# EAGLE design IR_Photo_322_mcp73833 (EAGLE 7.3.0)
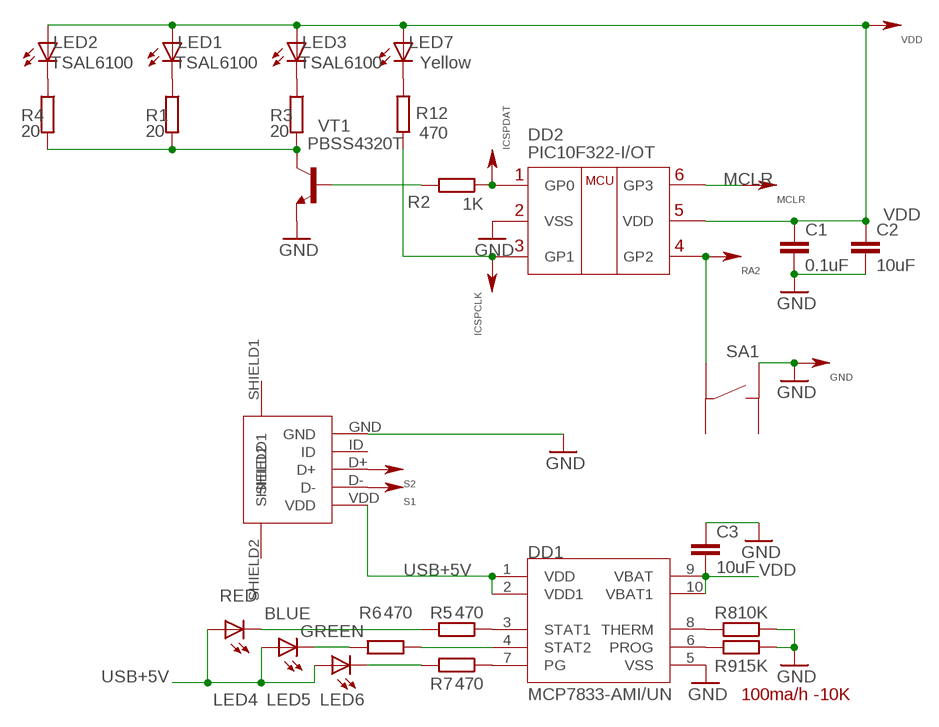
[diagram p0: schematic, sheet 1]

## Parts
C1  0.1uF  C-EUC0805  [C0805]
C2  10uF  C-EUC0805  [C0805]
C3  10uF  C-EUC0805  [C0805]
DD1  MCP7833-AMI/UN  MCP73833  [MSOP10]
DD2  PIC10F322-I/OT  PIC10F20XSOT23-6  [SOT23-6]
GND  1-PINSMD  [1-PINSMD]
ICSPCLK  1-PINSMD  [1-PINSMD]
ICSPDAT  1-PINSMD  [1-PINSMD]
LED1  TSAL6100  LEDNO_HOLE_MIR  [LED_NO_HOLE_MIR]
LED2  TSAL6100  LEDNO_HOLE_MIR  [LED_NO_HOLE_MIR]
LED3  TSAL6100  LEDNO_HOLE_MIR  [LED_NO_HOLE_MIR]
LED4  RED  LEDCHIPLED_1206  [CHIPLED_1206]
LED5  BLUE  LEDCHIPLED_1206  [CHIPLED_1206]
LED6  GREEN  LEDCHIPLED_1206  [CHIPLED_1206]
LED7  Yellow  LEDCHIPLED_1206  [CHIPLED_1206]
MCLR  1-PINSMD  [1-PINSMD]
R1  20  R-EU_R0805  [R0805]
R2  1K  R-EU_R0603  [R0603]
R3  20  R-EU_R0805  [R0805]
R4  20  R-EU_R0805  [R0805]
R5  470  R-EU_R0603  [R0603]
R6  470  R-EU_R0603  [R0603]
R7  470  R-EU_R0603  [R0603]
R8  10K  R-EU_R0603  [R0603]
R9  15K  R-EU_R0603  [R0603]
R12  470  R-EU_R0603  [R0603]
RA2  1-PINSMD  [1-PINSMD]
S1  1-PINSMD  [1-PINSMD]
S2  1-PINSMD  [1-PINSMD]
SA1  TACKT_BUTTONIIT-1102S  [IIT-1102S]
U$8  USB-MICRO  [USB-MICRO-SMD]
VDD  1-PINSMD  [1-PINSMD]
VT1  PBSS4320T  PBSS4320T-NPN-SOT23-BEC  [SOT23-BEC]

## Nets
GND: C1.2 C2.2 C3.1 DD1.5(VSS) DD2.2(VSS) GND.1(S) R8.1 R9.1 SA1.SR U$8.GND VT1.E
ICSPDAT: DD2.1(GP0) ICSPDAT.1(S) R2.1
MCLR: DD2.6(GP3) MCLR.1(S)
N$1: LED1.CATOD(C) R1.1
N$2: LED7.C R12.2
N$4: LED2.CATOD(C) R4.1
N$5: R2.2 VT1.B
N$6: R1.2 R3.2 R4.2 VT1.C
N$8: DD2.4(GP2) RA2.1(S) SA1.SSR
N$9: LED3.CATOD(C) R3.1
N$10: DD1.3(STAT1) R5.1
N$11: DD1.7(PG) R7.1
N$12: S1.1(S) U$8.D-
N$13: DD1.6(PROG) R9.2
N$14: LED4.C R5.2
N$15: LED5.C R6.2
N$16: DD1.4(STAT2) R6.1
N$17: LED6.C R7.2
N$18: DD1.8(THERM) R8.2
N$19: S2.1(S) U$8.D+
N$24: DD2.3(GP1) ICSPCLK.1(S) R12.1
USB+5V: DD1.1(VDD) DD1.2(VDD1) LED4.A LED5.A LED6.A U$8.VDD
VDD: C1.1 C2.1 C3.2 DD1.9(VBAT) DD1.10(VBAT1) DD2.5(VDD) LED1.ANOD(A) LED2.ANOD(A) LED3.ANOD(A) LED7.A VDD.1(S)
Unconnected: SA1.SL SA1.SSL U$8.ID U$8.SHIELD1 U$8.SHIELD2

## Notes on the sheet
- 100ma/h -10K

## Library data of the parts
C1-C3 = resistors:C-EU: CAPACITOR, European symbol
DD1 = power:MCP73833
DD2 = Microchip:PIC10F20X
GND ICSPCLK ICSPDAT MCLR RA2 S1 S2 VDD = connectors:1-PIN
LED1-LED7 = led:LED: LED
R1-R9 R12 = resistors:R-EU_: RESISTOR, European symbol
SA1 = button:TACKT_BUTTON
U$8 = connectors:USB-MICRO
VT1 = Tranzistors:*-NPN-: NPN Transistror BF959 corrected 2008.03.06

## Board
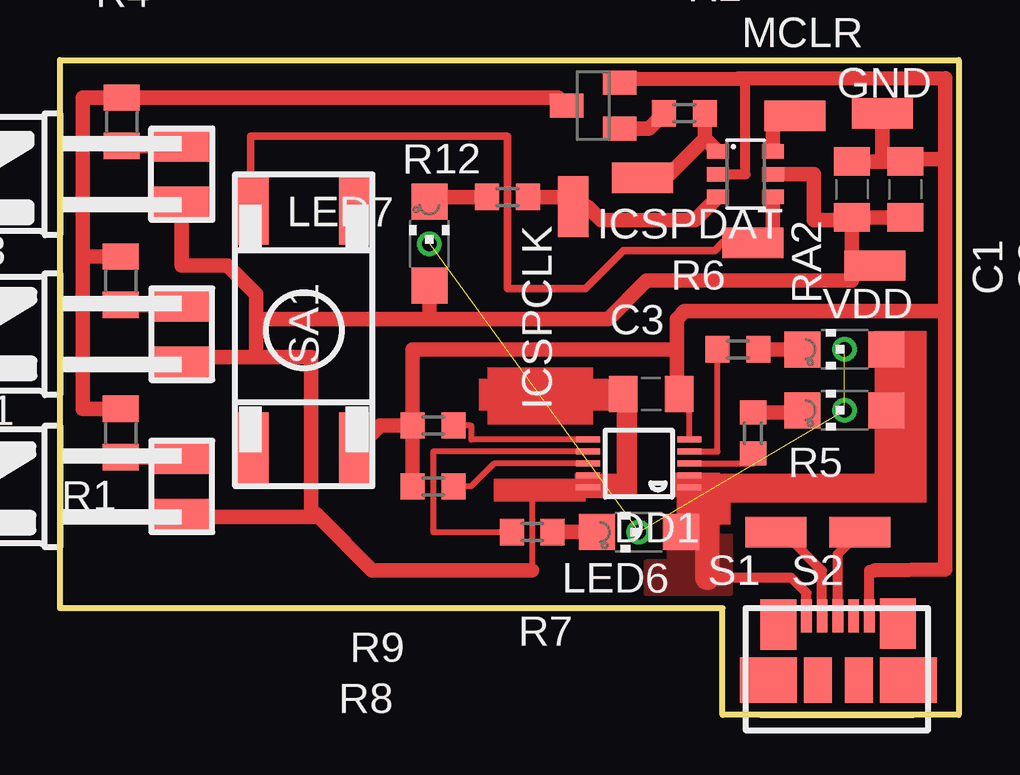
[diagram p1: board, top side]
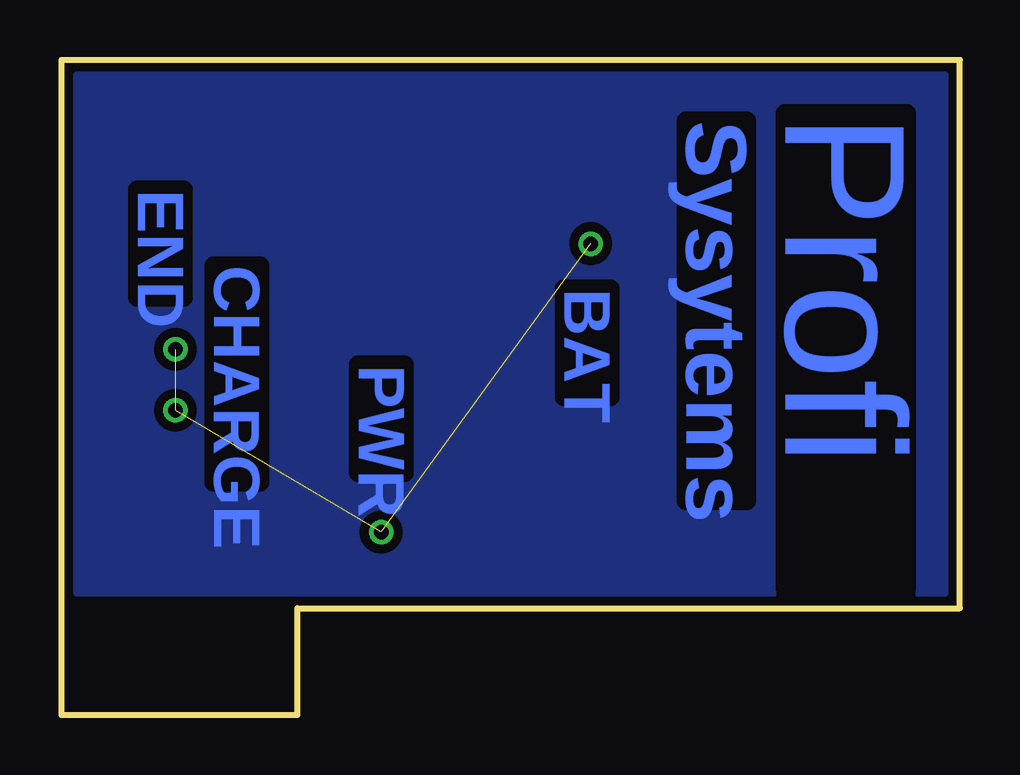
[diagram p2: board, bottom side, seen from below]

Size 37.47 x 27.3 mm. Coordinates in mm from the lower left corner, seen from the top.
Outline: 37.45,4.45 37.45,27.29 0,27.29 0,4.45
Outline: 0,4.45 27.62,4.45 27.62,0 37.47,0 37.47,27.3 0,27.3 0,4.45
Copper layers (1*16): Top 0.035mm / dielectric 1.5mm / Bottom 0.035mm
Design rules "default *": minimum track width 4mil, minimum drill 2mil, track to track 15mil, track to pad 8mil, pad to pad 8mil, via to via 8mil, smd to smd 8mil, copper to edge 10mil, drill to drill 20mil, minimum pad ring 4mil, minimum via ring 4mil, stop-mask expansion 4mil, vias tented up to drill 0mil, thermal gap 10mil

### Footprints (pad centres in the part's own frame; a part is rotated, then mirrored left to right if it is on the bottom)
C0805 = smd 1.2 x 1.5: 1 -1.167,0; 2 1.167,0
MSOP10 = smd 0.25 x 1: 1 -1,-2.113; 2 -0.5,-2.113; 3 0,-2.113; 4 0.5,-2.113; 5 1,-2.113; 6 1,2.113; 7 0.5,2.113; 8 0,2.113; 9 -0.5,2.113; 10 -1,2.113
SOT23-6 = smd 0.6 x 0.9: 1 -0.95,-1.15; 2 0,-1.15; 3 0.95,-1.15; 4 0.95,1.15; 5 0,1.15; 6 -0.95,1.15
1-PINSMD = smd 2.54 x 1.27: 1 0,0
LED_NO_HOLE_MIR = smd 2.5 x 1.5: ANOD 0,2.54; CATOD 0,0
CHIPLED_1206 = smd 1.5 x 1.5: A 0,-1.75; C 0,1.75
R0805 = smd 1.1 x 1.5: 1 -1.009,0; 2 1.009,0
R0603 = smd 1 x 1.1: 1 -0.85,0; 2 0.85,0
IIT-1102S = smd 3 x 1.5: SL 10.001,0; SR 0,0; SSL 0,4.445; SSR 10.001,4.445
USB-MICRO-SMD = smd 1.38 x 0.45: D+ 0,-1.627; D- 0,-0.972; GND 0,-2.937; ID 0,-2.282; VDD 0,-0.318 | smd 2.1 x 1.5: P$1 -0.318,-4.128; P$2 -0.357,0.853 | smd 1.9 x 1.175: P$5 -2.679,-2.5; P$6 -2.679,-0.794 | smd 1.9 x 2.375: SHIELD1 -2.679,1.27; SHIELD2 -2.679,-4.564
SOT23-BEC = smd 1 x 1.4: B -0.95,-1.1; C 0,1.1; E 0.95,-1.1

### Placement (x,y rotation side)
C1  33.02,21.91 90 top
C2  35.24,21.91 90 top
C3  24.65,13.37 180 top
DD1  24.13,10.48 90 top
DD2  28.57,22.54 270 top
GND  34.29,25.08 0 top
ICSPCLK  21.39,21.19 90 top
ICSPDAT  24.29,22.38 180 top
LED1  5.08,10.79 180 top
LED2  5.08,23.81 180 top
LED3  5.08,17.14 180 top
LED4  32.7,12.7 90 top
LED5  32.7,15.24 90 top
LED6  24.13,7.62 90 top
LED7  15.4,19.65 0 top
MCLR  30.64,24.96 0 top
R1  2.54,11.75 90 top
R2  26.04,25.08 180 top
R3  2.54,18.1 90 top
R4  2.58,24.73 90 top
R5  28.89,11.75 90 top
R6  28.26,15.24 0 top
R7  19.68,7.62 0 top
R8  15.56,9.53 0 top
R9  15.56,12.07 0 top
R12  18.65,21.59 180 top
RA2  28.89,19.69 180 top
S1  29.84,7.62 0 top
S2  33.34,7.62 0 top
SA1  12.38,11.11 90 top
U$8  30.8,4.13 90 top
VDD  33.97,18.73 180 top
VT1  22.23,25.4 90 top

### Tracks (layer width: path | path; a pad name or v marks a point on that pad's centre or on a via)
GND
  Top 0.254: DD1.5 26.24,12.95 C3.1
  Top 0.406: U$8.GND 33.73,6.03 33.97,6.03 | DD2.2 28.57,22.54 28.57,26.53
  Top 0.61: C1.2 34.29,23.07 | GND.1 34.29,23.07 | 34.29,23.07 C2.2 35.24,23.18 36.91,23.18 | R8.1 R9.1 | R9.1 13.34,12.07 SA1.SR | R9.1 14.71,15.24 25.72,15.24 | 25.72,15.24 25.72,13.38 C3.1 | VT1.E 23.32,26.51 28.26,26.53 28.57,26.53 36.91,26.55 36.91,23.18 | 36.91,23.18 36.91,16.83 | 36.91,16.83 36.91,6.07 33.97,6.03 | 25.72,15.24 25.72,16.51 26.04,16.83 36.91,16.83
ICSPDAT
  Top 0.61: R2.1 26.89,24.03 | 26.89,24.03 DD2.1 | 26.89,24.03 25.4,22.54 24.45,22.54 ICSPDAT.1
MCLR
  Top 0.61: DD2.6 29.73,24.96 MCLR.1
N$1
  Top 0.61: R1.1 5.08,10.74 LED1.CATOD
N$2
  Top 0.61: R12.2 15.59,21.59 LED7.C
N$4
  Top 0.61: 5.08,24.13 LED2.CATOD 5.08,23.72 R4.1
N$5
  Top 0.61: VT1.B 24.55,24.45 R2.2
N$6
  Top 0.61: R1.2 0.95,12.76 0.95,19.11 | 0.95,19.11 R3.2 | 0.95,19.11 0.95,25.73 R4.2 20.79,25.73 VT1.C
N$7  (via drill 0.6 pad 1.02)  (3 unrouted)
  other vias: 32.7,15.24 32.7,12.7 24.13,7.62 15.4,19.65
N$8
  Top 0.305: RA2.1 27.62,19.69 27.3,19.37 23.5,19.37 21.91,17.78 18.65,17.78 18.65,24.13 7.94,24.13 SA1.SSR
  Top 0.61: DD2.4 29.73,19.69 RA2.1
N$9
  Top 0.61: R3.1 5.08,17.09 LED3.CATOD
N$10
  Top 0.254: DD1.3 28.89,10.48 R5.1
N$11
  Top 0.254: DD1.7 15.56,10.98 15.56,7.62 R7.1
N$12
  Top 0.406: U$8.D- 31.77,6.01 30.32,7.46 S1.1
N$13
  Top 0.254: DD1.6 17.14,11.48 17.14,12.07 R9.2
N$14
  Top 0.61: 30.64,13.02 LED4.C 30.95,12.6 R5.2
N$15
  Top 0.61: R6.2 LED5.C
N$16
  Top 0.254: DD1.4 27.41,10.98 R6.1
N$17
  Top 0.61: R7.2 LED6.C
N$18
  Top 0.254: DD1.8 18.1,10.48 17.14,9.53 R8.2
N$19
  Top 0.406: U$8.D+ 32.42,6.71 S2.1
N$23
  pour Bottom: 0.64,26.67 36.83,26.67 36.83,5.08 0.64,5.08
N$24
  Top 0.406: 27.3,21.59 DD2.3
  Top 0.61: 27.3,21.59 | R12.1 21,21.59 ICSPCLK.1 21.99,21.19 22.54,20.64 26.47,20.64 DD2.3
USB+5V
  Top 0.254: DD1.1 DD1.2 | 26.99,9.48 26.99,9.53
  Top 0.406: U$8.VDD 31.11,5.08 30.48,5.71 26.99,5.71 | 26.24,9.53 DD1.1
  Top 0.61: LED5.A LED4.A 34.45,9.48 26.99,9.48 DD1.1 26.2,9.53 | LED6.A 26.99,7.62
  Top 1.016: 26.99,5.71 26.99,7.62 26.99,9.48
  pour Top (no thermals): 25.84,9.96 25.84,8.69 25.4,8.69 25.4,6.35 24.45,6.35 24.45,5.08 27.94,5.08 27.94,9.96
VDD
  Top 0.254: DD1.9 DD1.10 | DD1.10 19.68,9.48 19.68,6.03 | DD1.10 23.81,9.48 23.81,13.04 C3.2
  Top 0.305: LED2.ANOD 5.4,21.27
  Top 0.406: DD1.10 23.13,9.48 | 10.48,8.53 10.48,8.57
  Top 0.61: DD2.5 31.43,22.54 31.43,20.64 33.02,20.64 C1.1 | C2.1 C1.1 | 33.02,18.73 C1.1 | VDD.1 33.02,18.73 | 19.68,6.03 13.02,6.03 10.79,8.26 | 10.79,8.26 10.48,8.57 10.48,14.92 8.26,14.92 | LED1.ANOD 10.79,8.26 | LED3.ANOD arc-90 5.4,14.92 8.26,14.92 | 8.18,16.51 8.18,17.54 6.99,18.73 5.08,18.73 LED2.ANOD | 8.18,16.51 8.18,15 8.26,14.92 | 8.18,16.51 15.56,16.51 | 33.02,18.73 33.02,18.1 24.45,18.1 22.86,16.51 15.56,16.51 | LED7.A 15.4,16.67 15.56,16.51
(copper drawn outside any net)
  shapes: Top area x9

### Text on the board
Bottom: Profi | Sysytems | END | CHARGE | BAT | PWR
